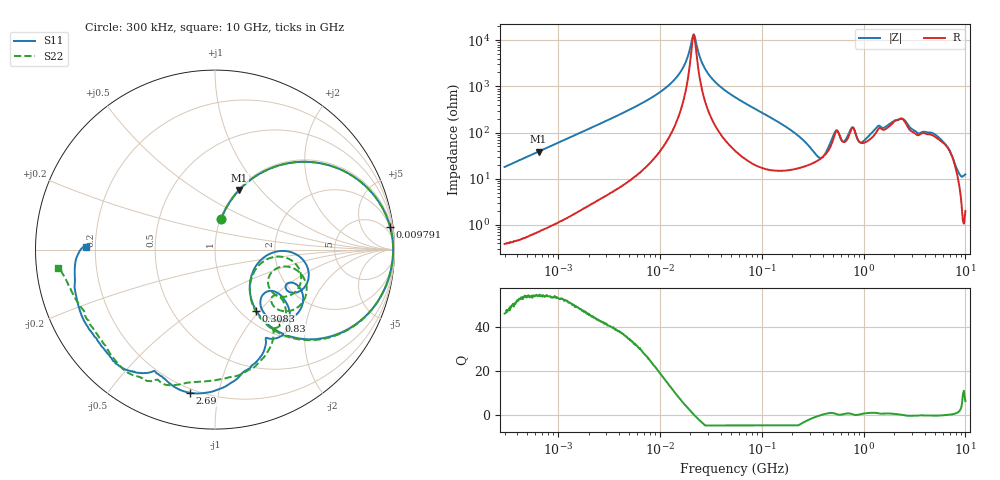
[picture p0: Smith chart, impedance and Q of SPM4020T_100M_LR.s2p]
! S-Parameter Data Generated by TDK Corporation
! Copyright(C) 2019 TDK Corporation.
! All Rights Reserved.
! TDK P/N: SPM4020T-100M-LR (Inductor)
! Property: L=10uH at 100kHz
! Size(LxWxT): 4.4x4.1x2mm
! Model Type: s2p (Touchstone File Format Version 1.0)
! Frequency: DC=Yes Start=0.3MHz Stop=10000MHz 802points Log-sweep
! Model Generated on Sep. 23, 2019
! Port Assignments:
!  1 ---@@@--- 2
! Applicable Conditions:
!  Temperature = 25 degC
!  DC Bias Current = 0 A
!  Small Signal Operation
! Terms and conditions regarding TDK Simulation Models
! (1)This simulation model is being provided solely for informational purposes. Please refer to the specifications of the products in terms of detailed characteristics of such products.
! (2)In no event shall TDK Corporation of any of its subsidiaries be liable for any loss or damage arising, directly or indirectly,
!  From any information contained in this simulation model, including, but not limited to loss or damages arising from any inaccuracies, omissions or errors in connection with such information.
! (3)Any and all copyrights on this simulation model are owned by TDK Corporation.
!  Duplication or redistribution of this simulation model without prior written permission from TDK Corporation is prohibited.
! (4)This simulation model is subject to any modification or change without any prior notice.
! (5)Neither TDK Corporation nor any of its subsidiaries shall make any warranty, express or implied,
!  Including but not limited to the correctness, implied warranties of merchantability and fitness for a particular purpose with respect to this simulation models.
! (6)The use of this simulation model shall be deemed to have consented to the terms and conditions hereof.
# Hz S MA R 50
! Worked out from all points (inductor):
!   801 points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, 300 kHz to 10 GHz, reference 50 ohm
!   read as one part in series: L = 9.55 uH near 318.3 kHz
!   highest Q = 54.6 at 645.5 kHz (marker M1), where L = 9.56 uH
!   self-resonance near 21.26 MHz
!   S11 on the Smith chart (normalised r, x): 300 kHz: 1.01, +0.36; 9.791 MHz: 2, +15; 308.3 MHz: 1.17, -0.96; 830 MHz: 1.25, -1.39; 2.69 GHz: 0.18, -0.83; 10 GHz: 0.17, +0.01
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300000  0.1764 78.6  0.9806 -10.2  0.9804 -10.2  0.1762 78.5
645490  0.3589 67.9  0.9268 -21.1  0.9268 -21.1  0.3588 67.9
1713600  0.7085 43.7  0.6911 -45.1  0.6911 -45.2  0.7085 43.7
9671944  0.9834 7.6  0.1389 -79.5  0.139 -79.5  0.9834 7.6
9790704  0.9838 7.5  0.1365 -79.6  0.1365 -79.6  0.9837 7.5
1.603896e7  0.9919 2.1  0.04768 -79.5  0.0477 -79.5  0.9919 2.1
2.15778e7  0.9925 -0.8  0.00746 -0.1  0.00747 -0.1  0.9925 -0.8
2.856806e7  0.9907 -3.6  0.04534 75.9  0.04537 75.9  0.9907 -3.7
5.477226e7  0.9746 -11.6  0.1663 74.4  0.1664 74.4  0.9746 -11.7
1.720721e8  0.7768 -39.5  0.5519 44.1  0.5519 44.1  0.7763 -40.0
3.08327e8  0.4105 -56.0  0.7633 10.5  0.7634 10.5  0.4099 -56.5
3.126428e8  0.3994 -55.9  0.7658 9.5  0.7658 9.5  0.3989 -56.4
4.030213e8  0.2438 -28.9  0.7584 -10.6  0.7584 -10.6  0.251 -29.8
4.807079e8  0.3729 -1.1  0.6369 -26.6  0.6369 -26.6  0.3797 -6.1
5.414944e8  0.5392 -14.2  0.4666 -23.0  0.4667 -23.1  0.5127 -22.2
6.490631e8  0.442 -26.3  0.5991 -23.6  0.5991 -23.6  0.3364 -24.5
8.299813e8  0.5344 -48.0  0.465 -17.6  0.465 -17.6  0.5539 -36.9
1.10164e9  0.4077 -35.1  0.5576 -46.4  0.5576 -46.4  0.4398 -36.3
1.767019e9  0.6048 -62.3  0.3318 -68.4  0.3318 -68.4  0.626 -60.7
2.69003e9  0.8098 -99.8  0.2118 -54.0  0.2118 -54.0  0.7458 -98.6
6.091595e9  0.8322 -136.4  0.1857 -88.0  0.1859 -88.1  0.8175 -137.6
1e10  0.7165 179.1  0.1163 -125.9  0.1164 -126.1  0.8815 -173.2
